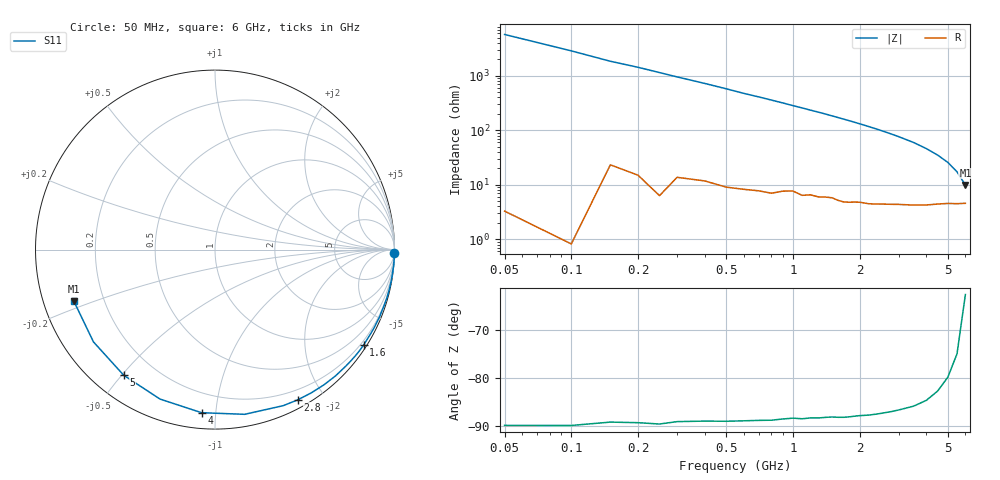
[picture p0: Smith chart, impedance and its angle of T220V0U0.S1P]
! SIEMENS Discrete & RF Semiconductors
! BAS70-04W
! Si Schottky Diode in SOT323
! VR = 20 V
! S-Parameters:  November  1997
# GHz  S  MA  R  50
!  f  S11
! GHz  MAG  ANG
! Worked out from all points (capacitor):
!   34 points, 50 MHz to 6 GHz, reference 50 ohm
!   read as one part to ground: C = 556 fF near 50 MHz
!   lowest |Z| = 9.86 ohm at 6 GHz (marker M1)
!   S11 on the Smith chart (normalised r, x): 50 MHz: open; 1.6 GHz: 0.10, -3.42; 2.8 GHz: 0.09, -1.69; 4 GHz: 0.09, -0.92; 5 GHz: 0.09, -0.51; 6 GHz: 0.09, -0.17
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0.05  1 -1.0
0.1  1 -2.0
0.15  0.9993 -3.1
0.2  0.9993 -4.0
0.25  0.9995 -5.0
0.4  0.9978 -7.9
0.5  0.9973 -9.9
0.6  0.9964 -12.0
0.8  0.9947 -15.9
1.1  0.9907 -22.0
1.2  0.9887 -24.1
1.3  0.9878 -26.1
1.4  0.986 -28.2
1.6  0.9838 -32.6
1.7  0.9829 -34.8
1.8  0.9809 -37.0
2  0.9761 -41.6
2.2  0.9727 -46.3
2.4  0.9676 -51.1
2.6  0.9617 -56.1
2.8  0.9556 -61.2
3  0.949 -66.4
3.5  0.9325 -79.8
4  0.9118 -94.7
4.5  0.8874 -110.2
5  0.8653 -126.0
5.5  0.8503 -142.8
6  0.8374 -160.0
